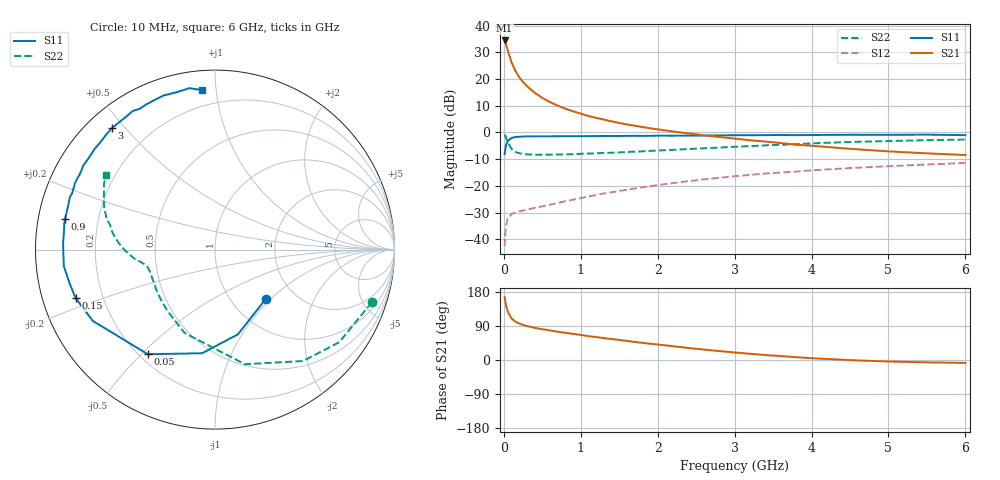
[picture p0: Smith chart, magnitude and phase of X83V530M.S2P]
! SIEMENS Small Signal Semiconductors
! BFP136W
! Si NPN RF Bipolar Junction Transistor in SOT343
! VCE = 3.5 V  IC = 30 mA
! Common Emitter S-Parameters:  September  1994
# GHz  S  MA  R  50
!  f  S11  S21  S12  S22
! GHz  MAG  ANG  MAG  ANG  MAG  ANG  MAG  ANG
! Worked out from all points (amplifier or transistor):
!   40 points, 10 MHz to 6 GHz, reference 50 ohm
!   highest |S21| = 34.5 dB at 10 MHz (marker M1)
!   |S21| within 3 dB of that: start of sweep to 43.31 MHz
!   unconditionally stable (mu >= 1): 779.7 MHz to 2.786 GHz
!   at 200 MHz: K = 0.42, MSG = 25.1 dB, |S12| = -29.5 dB
!   at 1.5 GHz: K = 1.14, MAG = 10.5 dB, |S12| = -21.9 dB
!   at 6 GHz: K = 0.98, MSG = 1.5 dB, |S12| = -11.4 dB
!   S11 on the Smith chart (normalised r, x): 10 MHz: 1.43, -0.93; 50 MHz: 0.23, -0.52; 150 MHz: 0.10, -0.17; 900 MHz: 0.08, +0.10; 3 GHz: 0.07, +0.46; 6 GHz: 0.11, +0.92
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0.01  0.3946 -44.3  52.96 166.1  0.0074 74.2  0.9216 -18.6
0.02  0.4893 -74.9  48.55 153.3  0.0134 65.5  0.8631 -36.7
0.03  0.582 -97.1  44.14 143.0  0.0183 55.8  0.7912 -51.7
0.05  0.6928 -122.7  34.54 127.8  0.0242 43.2  0.6599 -75.4
0.1  0.7881 -149.7  20.64 109.7  0.0295 31.3  0.4944 -110.0
0.15  0.822 -160.7  14.35 101.2  0.0317 29.1  0.4323 -128.0
0.2  0.8314 -166.9  10.87 96.1  0.0334 28.2  0.4076 -138.8
0.25  0.8399 -171.1  8.793 92.4  0.0344 29.4  0.3961 -145.8
0.3  0.8473 -173.8  7.375 89.7  0.0357 30.3  0.388 -150.6
0.4  0.845 -178.8  5.562 85.0  0.0387 33.9  0.3836 -156.9
0.5  0.8471 177.7  4.436 81.2  0.0412 37.0  0.3826 -160.9
0.6  0.8467 175.2  3.699 78.0  0.0442 39.9  0.3841 -163.1
0.7  0.8486 172.2  3.187 74.6  0.0476 43.0  0.3864 -164.6
0.9  0.8525 168.3  2.492 68.9  0.055 46.4  0.3924 -167.1
1.1  0.8536 163.8  2.034 62.9  0.063 49.7  0.4024 -168.4
1.5  0.8586 156.7  1.506 52.9  0.0801 52.9  0.4233 -170.9
2.2  0.869 144.3  1.044 36.3  0.1125 52.7  0.4723 -176.1
3  0.8873 130.3  0.767 19.9  0.1513 48.1  0.5385 176.0
3.2  0.8881 126.9  0.715 16.4  0.1602 46.5  0.5547 173.7
4.5  0.9054 108.4  0.494 -0.4  0.2152 35.2  0.6631 158.8
5.5  0.9107 99.0  0.406 -6.2  0.251 27.2  0.7173 149.6
6  0.8906 94.5  0.378 -7.6  0.2684 22.7  0.7368 145.8
